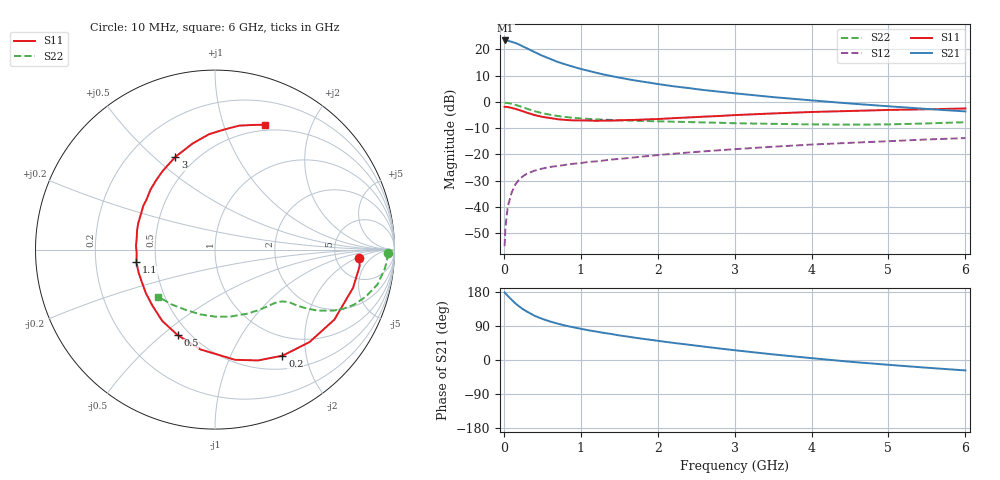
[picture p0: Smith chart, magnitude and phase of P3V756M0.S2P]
! SIEMENS Small Signal Semiconductors
! BFP181
! Si NPN RF Bipolar Junction Transistor in SOT143
! VCE = 0.75 V  IC = 6 mA
! Common Emitter S-Parameters:  March  1996
# GHz  S  MA  R  50
!  f  S11  S21  S12  S22
! GHz  MAG  ANG  MAG  ANG  MAG  ANG  MAG  ANG
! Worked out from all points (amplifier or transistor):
!   36 points, 10 MHz to 6 GHz, reference 50 ohm
!   highest |S21| = 23.4 dB at 20 MHz (marker M1)
!   |S21| within 3 dB of that: start of sweep to 301.1 MHz
!   unconditionally stable (mu >= 1): 958.7 MHz to end of sweep
!   at 250 MHz: K = 0.34, MSG = 24.7 dB, |S12| = -28.2 dB
!   at 1.4 GHz: K = 1.23, MAG = 13.0 dB, |S12| = -21.9 dB
!   at 6 GHz: K = 1.24, MAG = 2.1 dB, |S12| = -13.8 dB
!   S11 on the Smith chart (normalised r, x): 10 MHz: 8.72, -2.24; 200 MHz: 0.69, -1.60; 500 MHz: 0.43, -0.56; 1.1 GHz: 0.39, -0.07; 3 GHz: 0.39, +0.59; 6 GHz: 0.44, +1.39
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0.01  0.8058 -3.2  14.71 178.1  0.0018 83.2  0.9643 -1.2
0.02  0.8112 -6.5  14.78 176.2  0.004 82.6  0.9621 -2.5
0.05  0.7981 -15.5  14.64 169.3  0.01 83.0  0.9529 -6.3
0.1  0.771 -30.4  13.92 159.3  0.0186 73.1  0.9254 -12.2
0.15  0.7367 -44.4  13.24 149.5  0.0269 66.5  0.88 -17.3
0.2  0.7005 -57.6  12.35 141.3  0.0336 61.5  0.8338 -21.6
0.25  0.6622 -68.8  11.33 133.9  0.0388 56.4  0.7868 -24.8
0.3  0.6241 -79.7  10.48 127.8  0.0431 52.8  0.742 -27.3
0.4  0.5621 -98.3  8.876 116.6  0.0493 47.2  0.6654 -30.7
0.5  0.5199 -113.6  7.567 108.5  0.054 43.2  0.6105 -32.6
0.6  0.494 -126.6  6.617 101.7  0.0579 41.2  0.5707 -33.8
0.7  0.4683 -138.0  5.771 95.9  0.0604 39.9  0.5398 -34.6
0.9  0.4459 -156.1  4.678 86.5  0.0665 38.9  0.4992 -35.8
1.1  0.4433 -170.9  3.905 78.4  0.0721 38.4  0.4757 -37.4
1.5  0.4467 166.5  2.903 64.9  0.0825 38.4  0.4483 -41.4
1.8  0.4608 152.2  2.436 56.1  0.0912 38.0  0.4352 -45.4
2.2  0.4906 137.1  1.99 45.3  0.103 37.0  0.4205 -51.5
3  0.5614 113.2  1.459 25.8  0.1261 33.0  0.393 -66.5
3.5  0.6038 102.0  1.235 14.8  0.1406 30.3  0.3831 -77.7
4.5  0.6724 85.3  0.934 -4.6  0.1666 22.9  0.3703 -103.0
5.5  0.7249 73.3  0.735 -20.4  0.1931 16.3  0.3898 -128.4
6  0.7499 68.1  0.66 -27.5  0.2052 12.2  0.4111 -140.4
